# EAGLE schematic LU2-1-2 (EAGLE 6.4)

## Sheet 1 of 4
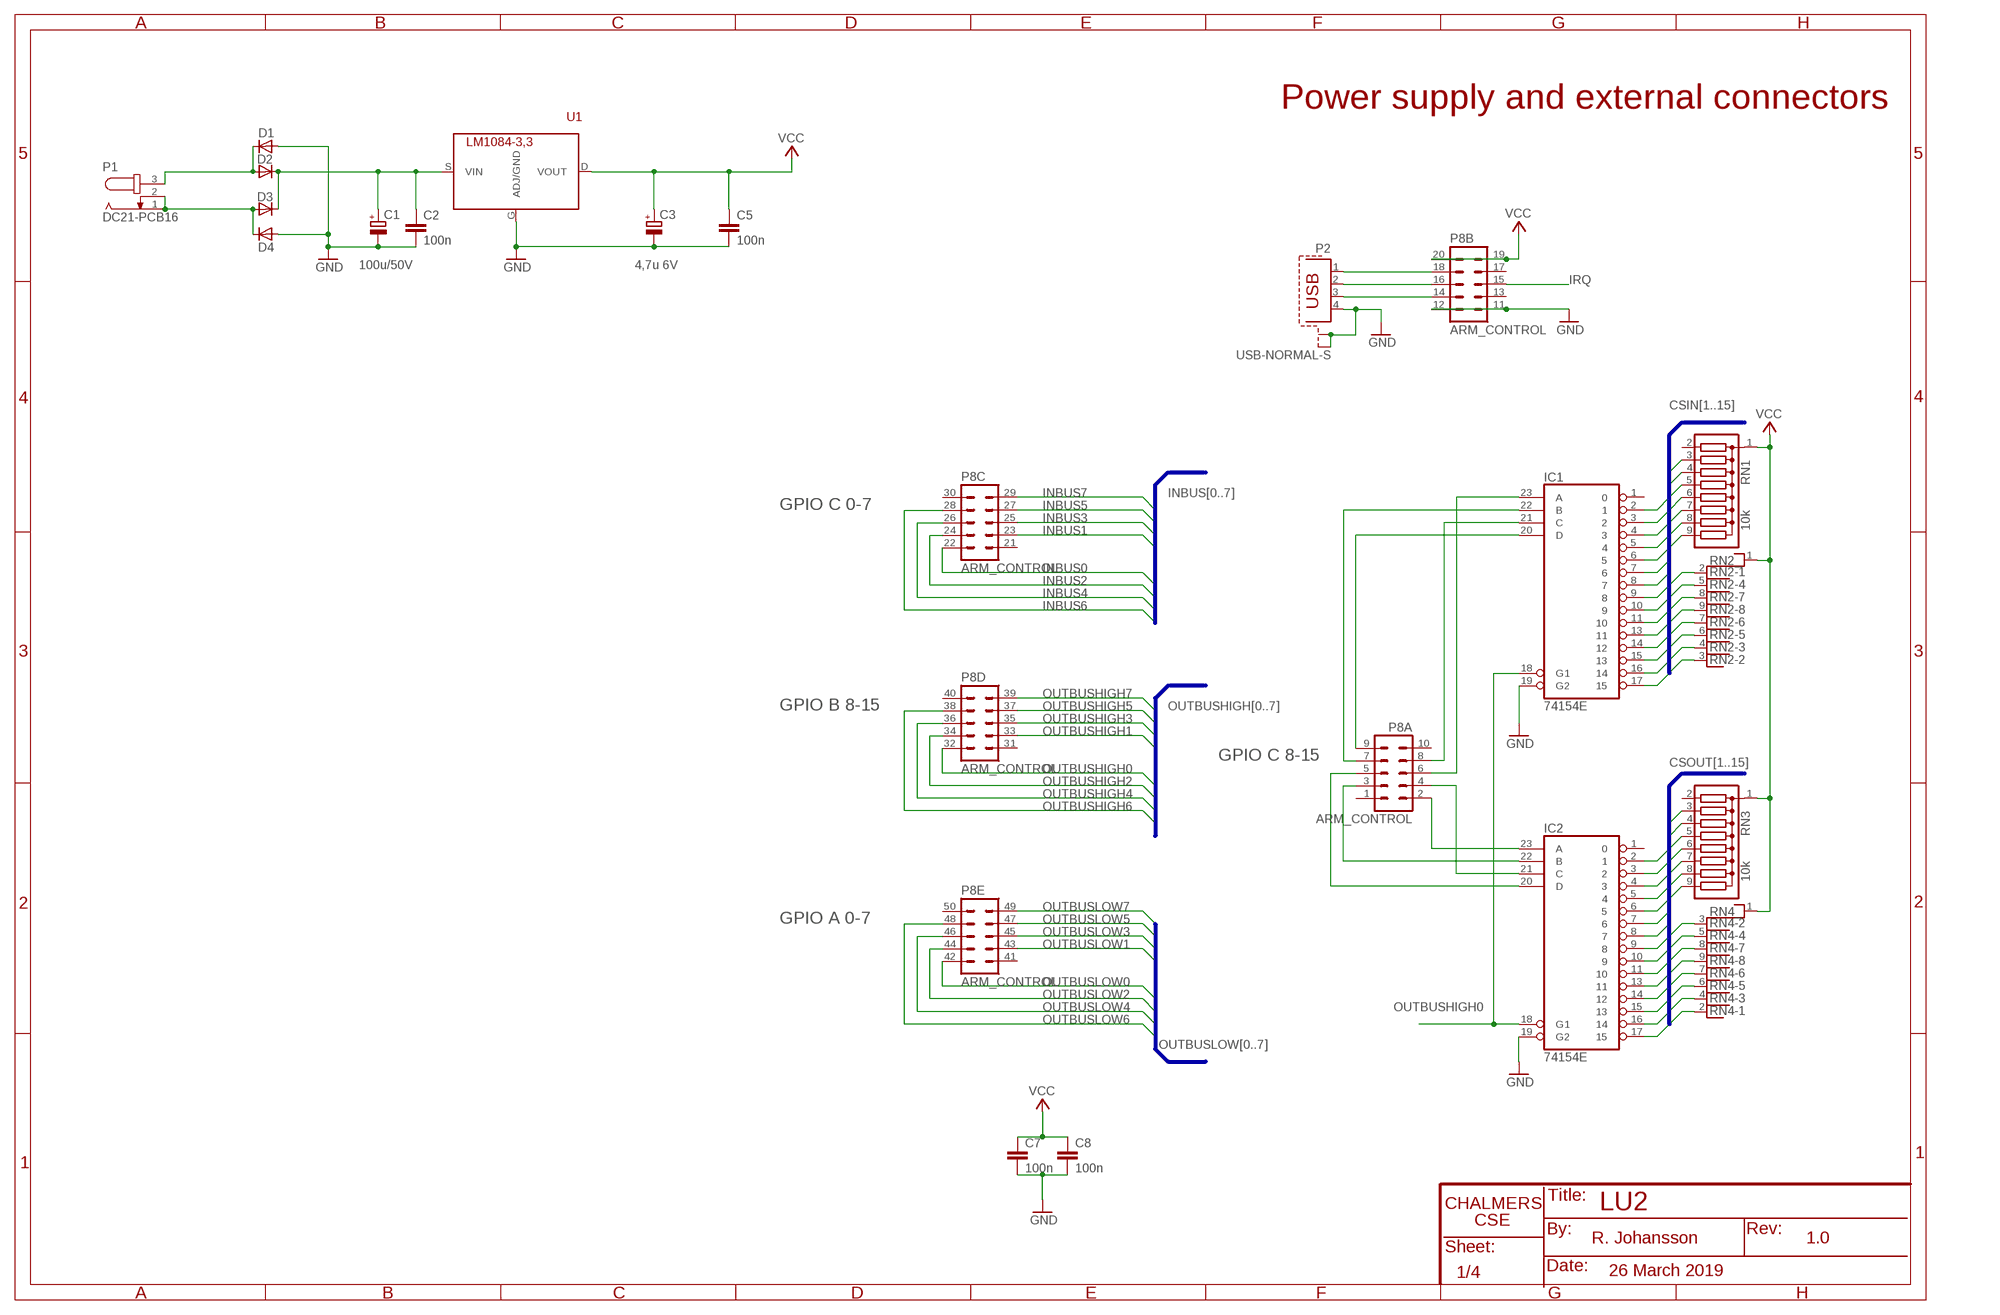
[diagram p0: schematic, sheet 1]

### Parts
C1  100u/50V  CPOL-EUE5-8.5  [E5-8,5]
C2  100n  C-EU050-024X044  [C050-024X044]
C3  4,7u 6V  CPOL-EUE5-5  [E5-5]
C5  100n  C-EU050-024X044  [C050-024X044]
C7  100n  C313  [C313]
C8  100n  C313  [C313]
D1  1N4004  [DO41-10]
D2  1N4004  [DO41-10]
D3  1N4004  [DO41-10]
D4  1N4004  [DO41-10]
IC1  74154E  [DIL24-3]
IC2  74154E  [DIL24-3]
P1  DC21-PCB16  [DC21CLIFF]
P2  USB-NORMAL-S  [1729-S]
P8  ARM_CONTROL  [ARM_CTRL]
RN1  10k  SIL9  [SIL9R]
RN2  RNX8  [RN-9]
RN3  10k  SIL9  [SIL9R]
RN4  RNX8  [RN-9]
U1  LM1084-3,3  LM1117T  [TO220AH]

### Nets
CSIN1: IC1.2 RN1.3 ; also sheet 4
CSIN2: IC1.3 RN1.4 ; also sheet 4
CSIN3: IC1.4 RN1.5 ; also sheet 4
CSIN4: IC1.5 RN1.6 ; also sheet 4
CSIN5: IC1.6 RN1.7 ; also sheet 3
CSIN6: IC1.7 RN1.8 ; also sheet 3
CSIN7: IC1.8 RN1.9 ; also sheet 3
CSIN8: IC1.9 RN2.2 ; also sheet 3
CSIN9: IC1.10 RN2.5 ; also sheet 2
CSIN10: IC1.11 RN2.8 ; also sheet 2
CSIN11: IC1.13 RN2.9
CSIN12: IC1.14 RN2.7
CSIN13: IC1.15 RN2.6
CSIN14: IC1.16 RN2.4
CSIN15: IC1.17 RN2.3
CSOUT1: IC2.2 RN3.3
CSOUT2: IC2.3 RN3.4
CSOUT3: IC2.4 RN3.5
CSOUT4: IC2.5 RN3.6
CSOUT5: IC2.6 RN3.7
CSOUT6: IC2.7 RN3.8
CSOUT7: IC2.8 RN3.9 ; also sheet 2
CSOUT8: IC2.9 RN4.3 ; also sheet 2
CSOUT9: IC2.10 RN4.5 ; also sheet 2
CSOUT10: IC2.11 RN4.8 ; also sheet 2
CSOUT11: IC2.13 RN4.9 ; also sheet 2
CSOUT12: IC2.14 RN4.7 ; also sheet 2
CSOUT13: IC2.15 RN4.6 ; also sheet 2
CSOUT14: IC2.16 RN4.4 ; also sheet 3
CSOUT15: IC2.17 RN4.2 ; also sheet 3
GND: C1.- C2.2 C3.- C5.2 C7.2 C8.2 D1.A D4.A IC1.19(G2) IC2.19(G2) P2.4 P2.S1 P2.S2 P8.11 P8.12 U1.G(ADJ/GND) ; also sheet 2,3,4
INBUS0: P8.22 ; also sheet 2,3
INBUS1: P8.23 ; also sheet 2,3
INBUS2: P8.24 ; also sheet 2,3
INBUS3: P8.25 ; also sheet 2,3
INBUS4: P8.26 ; also sheet 2,3
INBUS5: P8.27 ; also sheet 2,3
INBUS6: P8.28 ; also sheet 2,3
INBUS7: P8.29 ; also sheet 2,3
IRQ: P8.15 ; also sheet 3
N$29: IC1.21(C) P8.8
N$31: IC1.22(B) P8.7
N$33: IC1.23(A) P8.6
N$35: IC2.23(A) P8.2
N$37: IC2.22(B) P8.3
N$46: IC2.21(C) P8.4
N$47: IC2.20(D) P8.5
N$48: P2.1 P8.18
N$49: P2.2 P8.16
N$52: D3.A D4.C P1.1 P1.2
N$55: P2.3 P8.14
N$306: D1.C D2.A P1.3
N$307: C1.+ C2.1 D2.C D3.C U1.S(VIN)
N$342: IC1.20(D) P8.9
OUTBUSHIGH0: IC1.18(G1) IC2.18(G1) P8.32
OUTBUSHIGH1: P8.33 ; also sheet 2
OUTBUSHIGH2: P8.34 ; also sheet 4
OUTBUSHIGH3: P8.35 ; also sheet 4
OUTBUSHIGH4: P8.36 ; also sheet 4
OUTBUSHIGH5: P8.37 ; also sheet 4
OUTBUSHIGH6: P8.38
OUTBUSHIGH7: P8.39 ; also sheet 2
OUTBUSLOW0: P8.42 ; also sheet 2,3
OUTBUSLOW1: P8.43 ; also sheet 2,3
OUTBUSLOW2: P8.44 ; also sheet 2,3
OUTBUSLOW3: P8.45 ; also sheet 2,3
OUTBUSLOW4: P8.46 ; also sheet 2,3
OUTBUSLOW5: P8.47 ; also sheet 2,3
OUTBUSLOW6: P8.48 ; also sheet 2,3
OUTBUSLOW7: P8.49 ; also sheet 2,3
VCC: C3.+ C5.1 C7.1 C8.1 P8.19 P8.20 RN1.1 RN2.1 RN3.1 RN4.1 U1.D(VOUT) ; also sheet 2,3,4
Unconnected: IC1.1 IC2.1 P8.1 P8.10 P8.13 P8.17 P8.21 P8.30 P8.31 P8.40 P8.41 P8.50 RN1.2 RN3.2

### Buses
INBUS[0..7]
OUTBUSLOW[0..7]
OUTBUSHIGH[0..7]
CSOUT[1..15]
CSIN[1..15]

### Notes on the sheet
- Power supply and external connectors
- GPIO C 0-7
- GPIO B 8-15
- GPIO C 8-15
- GPIO A 0-7
- LU2
- 1.0
- R. Johansson
- 26 March 2019

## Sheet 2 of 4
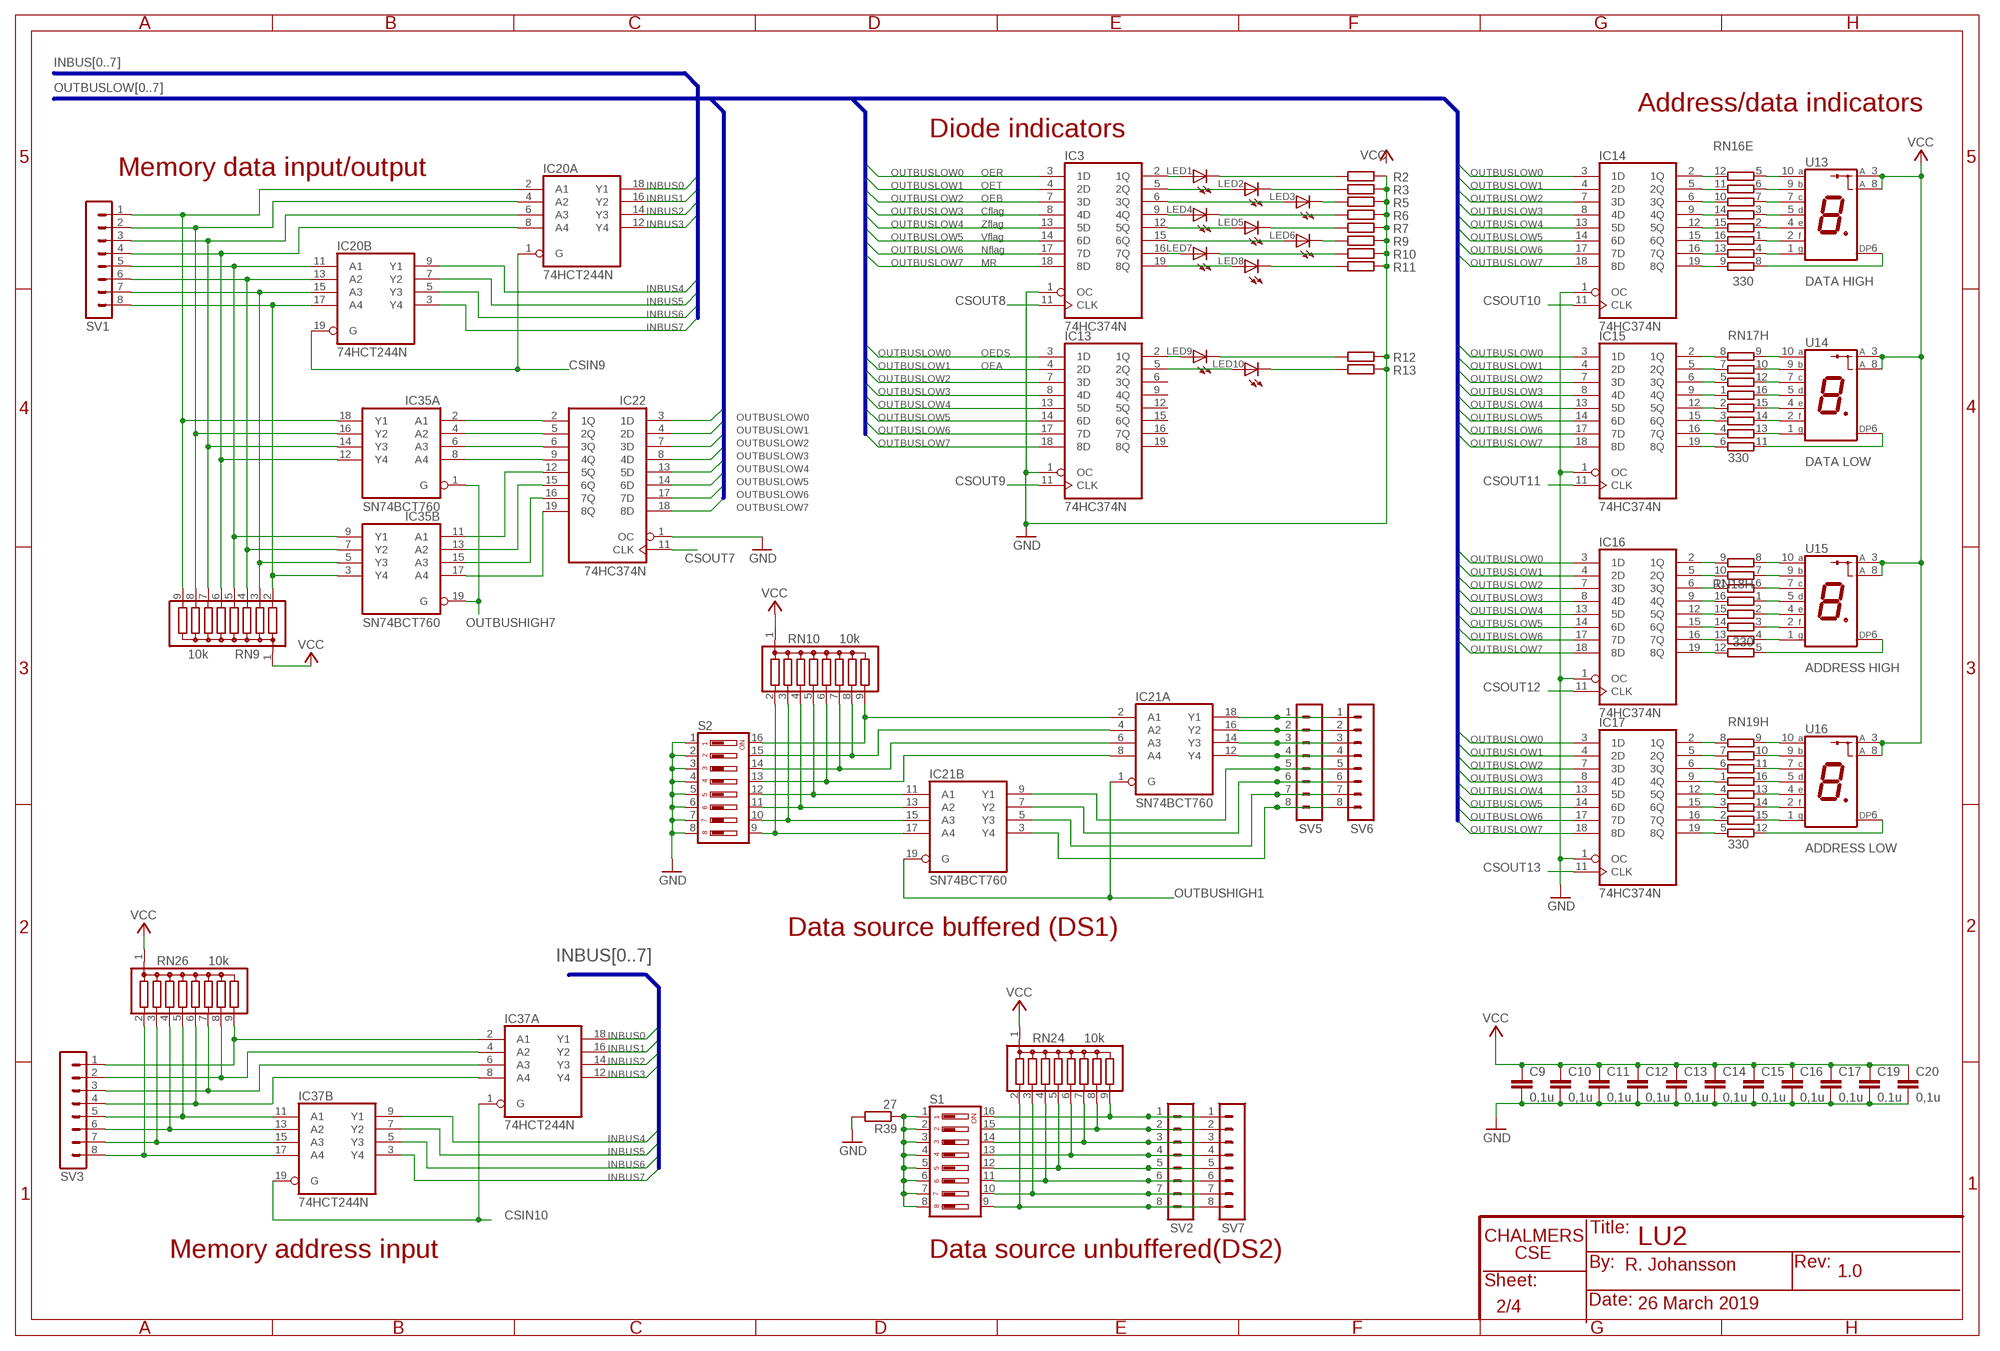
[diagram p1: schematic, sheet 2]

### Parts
C9  0,1u  C313  [C313]
C10  0,1u  C313  [C313]
C11  0,1u  C313  [C313]
C12  0,1u  C313  [C313]
C13  0,1u  C313  [C313]
C14  0,1u  C313  [C313]
C15  0,1u  C313  [C313]
C16  0,1u  C313  [C313]
C17  0,1u  C313  [C313]
C19  0,1u  C313  [C313]
C20  0,1u  C313  [C313]
IC3  74HC374N  [DIL20]
IC13  74HC374N  [DIL20]
IC14  74HC374N  [DIL20]
IC15  74HC374N  [DIL20]
IC16  74HC374N  [DIL20]
IC17  74HC374N  [DIL20]
IC20  74HCT244N  [DIL20]
IC21  SN74BCT760  74HCT244N  [DIL20]
IC22  74HC374N  [DIL20]
IC35  SN74BCT760  74HC244N  [DIL20]
IC37  74HCT244N  [DIL20]
LED1  RED  LED3MM  [LED3MM]
LED2  RED  LED3MM  [LED3MM]
LED3  RED  LED3MM  [LED3MM]
LED4  RED  LED3MM  [LED3MM]
LED5  RED  LED3MM  [LED3MM]
LED6  RED  LED3MM  [LED3MM]
LED7  RED  LED3MM  [LED3MM]
LED8  RED  LED3MM  [LED3MM]
LED9  RED  LED3MM  [LED3MM]
LED10  RED  LED3MM  [LED3MM]
R2  R-EU_0204/7  [0204/7]
R3  R-EU_0204/7  [0204/7]
R5  R-EU_0204/7  [0204/7]
R6  R-EU_0204/7  [0204/7]
R7  R-EU_0204/7  [0204/7]
R9  R-EU_0204/7  [0204/7]
R10  R-EU_0204/7  [0204/7]
R11  R-EU_0204/7  [0204/7]
R12  R-EU_0204/7  [0204/7]
R13  R-EU_0204/7  [0204/7]
R39  27  R-EU_0204/7  [0204/7]
RN9  10k  SIL9  [SIL9R]
RN10  10k  SIL9  [SIL9R]
RN16  330  8R-N  [DIL16]
RN17  330  8R-N  [DIL16]
RN18  330  8R-N  [DIL16]
RN19  330  8R-N  [DIL16]
RN24  10k  SIL9  [SIL9R]
RN26  10k  SIL9  [SIL9R]
S1  DS08  [DS-08]
S2  DS08  [DS-08]
SV1  MA08R-1  [MA08R-1]
SV2  MA08R-1  [MA08R-1]
SV3  MA08R-1  [MA08R-1]
SV5  MA08R-1  [MA08R-1]
SV6  MA08R-1  [MA08R-1]
SV7  MA08R-1  [MA08R-1]
U13  DATA HIGH  LED7_CA  [LED7SEG]
U14  DATA LOW  LED7_CA  [LED7SEG]
U15  ADDRESS HIGH  LED7_CA  [LED7SEG]
U16  ADDRESS LOW  LED7_CA  [LED7SEG]

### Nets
CSIN9: IC20.1(A:G) IC20.19(B:G) ; also sheet 1
CSIN10: IC37.1(A:G) IC37.19(B:G) ; also sheet 1
CSOUT7: IC22.11(CLK) ; also sheet 1
CSOUT8: IC3.11(CLK) ; also sheet 1
CSOUT9: IC13.11(CLK) ; also sheet 1
CSOUT10: IC14.11(CLK) ; also sheet 1
CSOUT11: IC15.11(CLK) ; also sheet 1
CSOUT12: IC16.11(CLK) ; also sheet 1
CSOUT13: IC17.11(CLK) ; also sheet 1
GND: C9.2 C10.2 C11.2 C12.2 C13.2 C14.2 C15.2 C16.2 C17.2 C19.2 C20.2 IC3.1(OC) IC13.1(OC) IC14.1(OC) IC15.1(OC) IC16.1(OC) IC17.1(OC) IC22.1(OC) R2.2 R3.2 R5.2 R6.2 R7.2 R9.2 R10.2 R11.2 R12.2 R13.2 R39.2 S2.1 S2.2 S2.3 S2.4 S2.5 S2.6 S2.7 S2.8 ; also sheet 1,3,4
INBUS0: IC20.18(A:Y1) IC37.18(A:Y1) ; also sheet 1,3
INBUS1: IC20.16(A:Y2) IC37.16(A:Y2) ; also sheet 1,3
INBUS2: IC20.14(A:Y3) IC37.14(A:Y3) ; also sheet 1,3
INBUS3: IC20.12(A:Y4) IC37.12(A:Y4) ; also sheet 1,3
INBUS4: IC20.9(B:Y1) IC37.9(B:Y1) ; also sheet 1,3
INBUS5: IC20.7(B:Y2) IC37.7(B:Y2) ; also sheet 1,3
INBUS6: IC20.5(B:Y3) IC37.5(B:Y3) ; also sheet 1,3
INBUS7: IC20.3(B:Y4) IC37.3(B:Y4) ; also sheet 1,3
N$1: IC13.2(1Q) LED9.A
N$3: IC13.5(2Q) LED10.A
N$4: IC3.19(8Q) LED8.A
N$5: IC3.16(7Q) LED7.A
N$7: IC22.19(8Q) IC35.17(B:A4)
N$8: LED1.K(C) R2.1
N$9: LED2.K(C) R3.1
N$10: LED3.K(C) R5.1
N$11: LED4.K(C) R6.1
N$12: LED5.K(C) R7.1
N$13: LED6.K(C) R9.1
N$14: LED7.K(C) R10.1
N$15: LED8.K(C) R11.1
N$16: IC3.15(6Q) LED6.A
N$17: IC3.12(5Q) LED5.A
N$18: IC20.17(B:A4) IC35.3(B:Y4) RN9.2 SV1.8
N$19: IC3.9(4Q) LED4.A
N$20: IC3.6(3Q) LED3.A
N$21: IC3.5(2Q) LED2.A
N$22: IC3.2(1Q) LED1.A
N$23: LED9.K(C) R12.1
N$24: LED10.K(C) R13.1
N$39: IC20.15(B:A3) IC35.5(B:Y3) RN9.3 SV1.7
N$78: IC20.13(B:A2) IC35.7(B:Y2) RN9.4 SV1.6
N$145: RN19.12 U16.6(DP)
N$146: RN19.15 U16.1(G)
N$147: RN19.14 U16.2(F)
N$148: RN19.13 U16.4(E)
N$149: RN19.16 U16.5(D)
N$150: RN19.11 U16.7(C)
N$151: RN19.10 U16.9(B)
N$152: RN19.9 U16.10(A)
N$153: IC17.19(8Q) RN19.5
N$154: IC17.16(7Q) RN19.2
N$155: IC17.15(6Q) RN19.3
N$156: IC17.12(5Q) RN19.4
N$157: IC17.9(4Q) RN19.1
N$158: IC17.6(3Q) RN19.6
N$159: IC17.5(2Q) RN19.7
N$160: IC17.2(1Q) RN19.8
N$161: RN18.5 U15.6(DP)
N$162: RN18.4 U15.1(G)
N$163: RN18.3 U15.2(F)
N$164: RN18.2 U15.4(E)
N$165: RN18.1 U15.5(D)
N$166: RN18.6 U15.7(C)
N$167: RN18.7 U15.9(B)
N$168: RN18.8 U15.10(A)
N$169: IC16.2(1Q) RN18.9
N$170: IC16.5(2Q) RN18.10
N$171: IC16.6(3Q) RN18.11
N$172: IC16.9(4Q) RN18.16
N$173: IC16.12(5Q) RN18.15
N$174: IC16.15(6Q) RN18.14
N$175: IC16.16(7Q) RN18.13
N$176: IC16.19(8Q) RN18.12
N$177: RN17.11 U14.6(DP)
N$178: RN17.13 U14.1(G)
N$179: RN17.14 U14.2(F)
N$180: RN17.15 U14.4(E)
N$181: RN17.16 U14.5(D)
N$182: RN17.12 U14.7(C)
N$183: RN17.10 U14.9(B)
N$184: RN17.9 U14.10(A)
N$185: IC15.19(8Q) RN17.6
N$186: IC15.16(7Q) RN17.4
N$187: IC15.15(6Q) RN17.3
N$188: IC15.12(5Q) RN17.2
N$189: IC15.9(4Q) RN17.1
N$190: IC15.6(3Q) RN17.5
N$191: IC15.5(2Q) RN17.7
N$192: IC15.2(1Q) RN17.8
N$197: IC14.2(1Q) RN16.12
N$198: IC14.5(2Q) RN16.11
N$199: IC14.6(3Q) RN16.10
N$200: IC14.9(4Q) RN16.14
N$201: IC14.12(5Q) RN16.15
N$202: IC14.15(6Q) RN16.16
N$203: IC14.16(7Q) RN16.13
N$204: IC14.19(8Q) RN16.9
N$213: RN16.5 U13.10(A)
N$214: RN16.6 U13.9(B)
N$215: RN16.7 U13.7(C)
N$216: RN16.3 U13.5(D)
N$217: RN16.2 U13.4(E)
N$218: RN16.1 U13.2(F)
N$219: RN16.4 U13.1(G)
N$220: RN16.8 U13.6(DP)
N$230: IC20.11(B:A1) IC35.9(B:Y1) RN9.5 SV1.5
N$248: IC20.8(A:A4) IC35.12(A:Y4) RN9.6 SV1.4
N$283: IC20.6(A:A3) IC35.14(A:Y3) RN9.7 SV1.3
N$284: IC20.4(A:A2) IC35.16(A:Y2) RN9.8 SV1.2
N$285: IC20.2(A:A1) IC35.18(A:Y1) RN9.9 SV1.1
N$287: IC21.17(B:A4) RN10.2 S2.9
N$288: IC21.15(B:A3) RN10.3 S2.10
N$289: IC21.13(B:A2) RN10.4 S2.11
N$290: IC21.11(B:A1) RN10.5 S2.12
N$291: IC21.8(A:A4) RN10.6 S2.13
N$292: IC21.6(A:A3) RN10.7 S2.14
N$293: IC21.4(A:A2) RN10.8 S2.15
N$294: IC21.2(A:A1) RN10.9 S2.16
N$358: IC22.16(7Q) IC35.15(B:A3)
N$359: IC22.15(6Q) IC35.13(B:A2)
N$360: IC22.12(5Q) IC35.11(B:A1)
N$361: IC22.9(4Q) IC35.8(A:A4)
N$362: IC22.6(3Q) IC35.6(A:A3)
N$363: IC22.5(2Q) IC35.4(A:A2)
N$364: IC22.2(1Q) IC35.2(A:A1)
N$381: R39.1 S1.1 S1.2 S1.3 S1.4 S1.5 S1.6 S1.7 S1.8
N$382: RN24.2 S1.9 SV2.8 SV7.8
N$383: RN24.3 S1.10 SV2.7 SV7.7
N$384: RN24.4 S1.11 SV2.6 SV7.6
N$385: RN24.5 S1.12 SV2.5 SV7.5
N$387: RN24.7 S1.14 SV2.3 SV7.3
N$388: RN24.8 S1.15 SV2.2 SV7.2
N$397: IC37.17(B:A4) RN26.2 SV3.8
N$406: IC37.15(B:A3) RN26.3 SV3.7
N$407: IC37.13(B:A2) RN26.4 SV3.6
N$408: IC37.11(B:A1) RN26.5 SV3.5
N$409: IC37.8(A:A4) RN26.6 SV3.4
N$412: IC37.6(A:A3) RN26.7 SV3.3
N$413: IC37.4(A:A2) RN26.8 SV3.2
N$419: RN24.9 S1.16 SV2.1 SV7.1
N$420: RN24.6 S1.13 SV2.4 SV7.4
N$436: IC37.2(A:A1) RN26.9 SV3.1
OUTBUSHIGH1: IC21.1(A:G) IC21.19(B:G) ; also sheet 1
OUTBUSHIGH7: IC35.1(A:G) IC35.19(B:G) ; also sheet 1
OUTBUSLOW0: IC3.3(1D) IC13.3(1D) IC14.3(1D) IC15.3(1D) IC16.3(1D) IC17.3(1D) IC22.3(1D) ; also sheet 1,3
OUTBUSLOW1: IC3.4(2D) IC13.4(2D) IC14.4(2D) IC15.4(2D) IC16.4(2D) IC17.4(2D) IC22.4(2D) ; also sheet 1,3
OUTBUSLOW2: IC3.7(3D) IC13.7(3D) IC14.7(3D) IC15.7(3D) IC16.7(3D) IC17.7(3D) IC22.7(3D) ; also sheet 1,3
OUTBUSLOW3: IC3.8(4D) IC13.8(4D) IC14.8(4D) IC15.8(4D) IC16.8(4D) IC17.8(4D) IC22.8(4D) ; also sheet 1,3
OUTBUSLOW4: IC3.13(5D) IC13.13(5D) IC14.13(5D) IC15.13(5D) IC16.13(5D) IC17.13(5D) IC22.13(5D) ; also sheet 1,3
OUTBUSLOW5: IC3.14(6D) IC13.14(6D) IC14.14(6D) IC15.14(6D) IC16.14(6D) IC17.14(6D) IC22.14(6D) ; also sheet 1,3
OUTBUSLOW6: IC3.17(7D) IC13.17(7D) IC14.17(7D) IC15.17(7D) IC16.17(7D) IC17.17(7D) IC22.17(7D) ; also sheet 1,3
OUTBUSLOW7: IC3.18(8D) IC13.18(8D) IC14.18(8D) IC15.18(8D) IC16.18(8D) IC17.18(8D) IC22.18(8D) ; also sheet 1,3
OUTBUSLOW8: IC21.18(A:Y1) SV5.1 SV6.1
OUTBUSLOW9: IC21.16(A:Y2) SV5.2 SV6.2
OUTBUSLOW10: IC21.14(A:Y3) SV5.3 SV6.3
OUTBUSLOW11: IC21.12(A:Y4) SV5.4 SV6.4
OUTBUSLOW12: IC21.9(B:Y1) SV5.5 SV6.5
OUTBUSLOW13: IC21.7(B:Y2) SV5.6 SV6.6
OUTBUSLOW14: IC21.5(B:Y3) SV5.7 SV6.7
OUTBUSLOW15: IC21.3(B:Y4) SV5.8 SV6.8
VCC: C9.1 C10.1 C11.1 C12.1 C13.1 C14.1 C15.1 C16.1 C17.1 C19.1 C20.1 RN9.1 RN10.1 RN24.1 RN26.1 U13.3(A) U13.8(A) U14.3(A) U14.8(A) U15.3(A) U15.8(A) U16.3(A) U16.8(A) ; also sheet 1,3,4
Unconnected: IC13.6(3Q) IC13.9(4Q) IC13.12(5Q) IC13.15(6Q) IC13.16(7Q) IC13.19(8Q)

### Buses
OUTBUSLOW[0..7]
INBUS[0..7]

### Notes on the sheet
- Address/data indicators
- Diode indicators
- Memory data input/output | OER
- OET
- OEB
- Cflag
- Zflag
- Vflag
- Nflag
- MR
- OEDS
- OEA
- Data source buffered (DS1)
- LU2
- Memory address input | Data source unbuffered(DS2)
- R. Johansson
- 1.0
- 26 March 2019

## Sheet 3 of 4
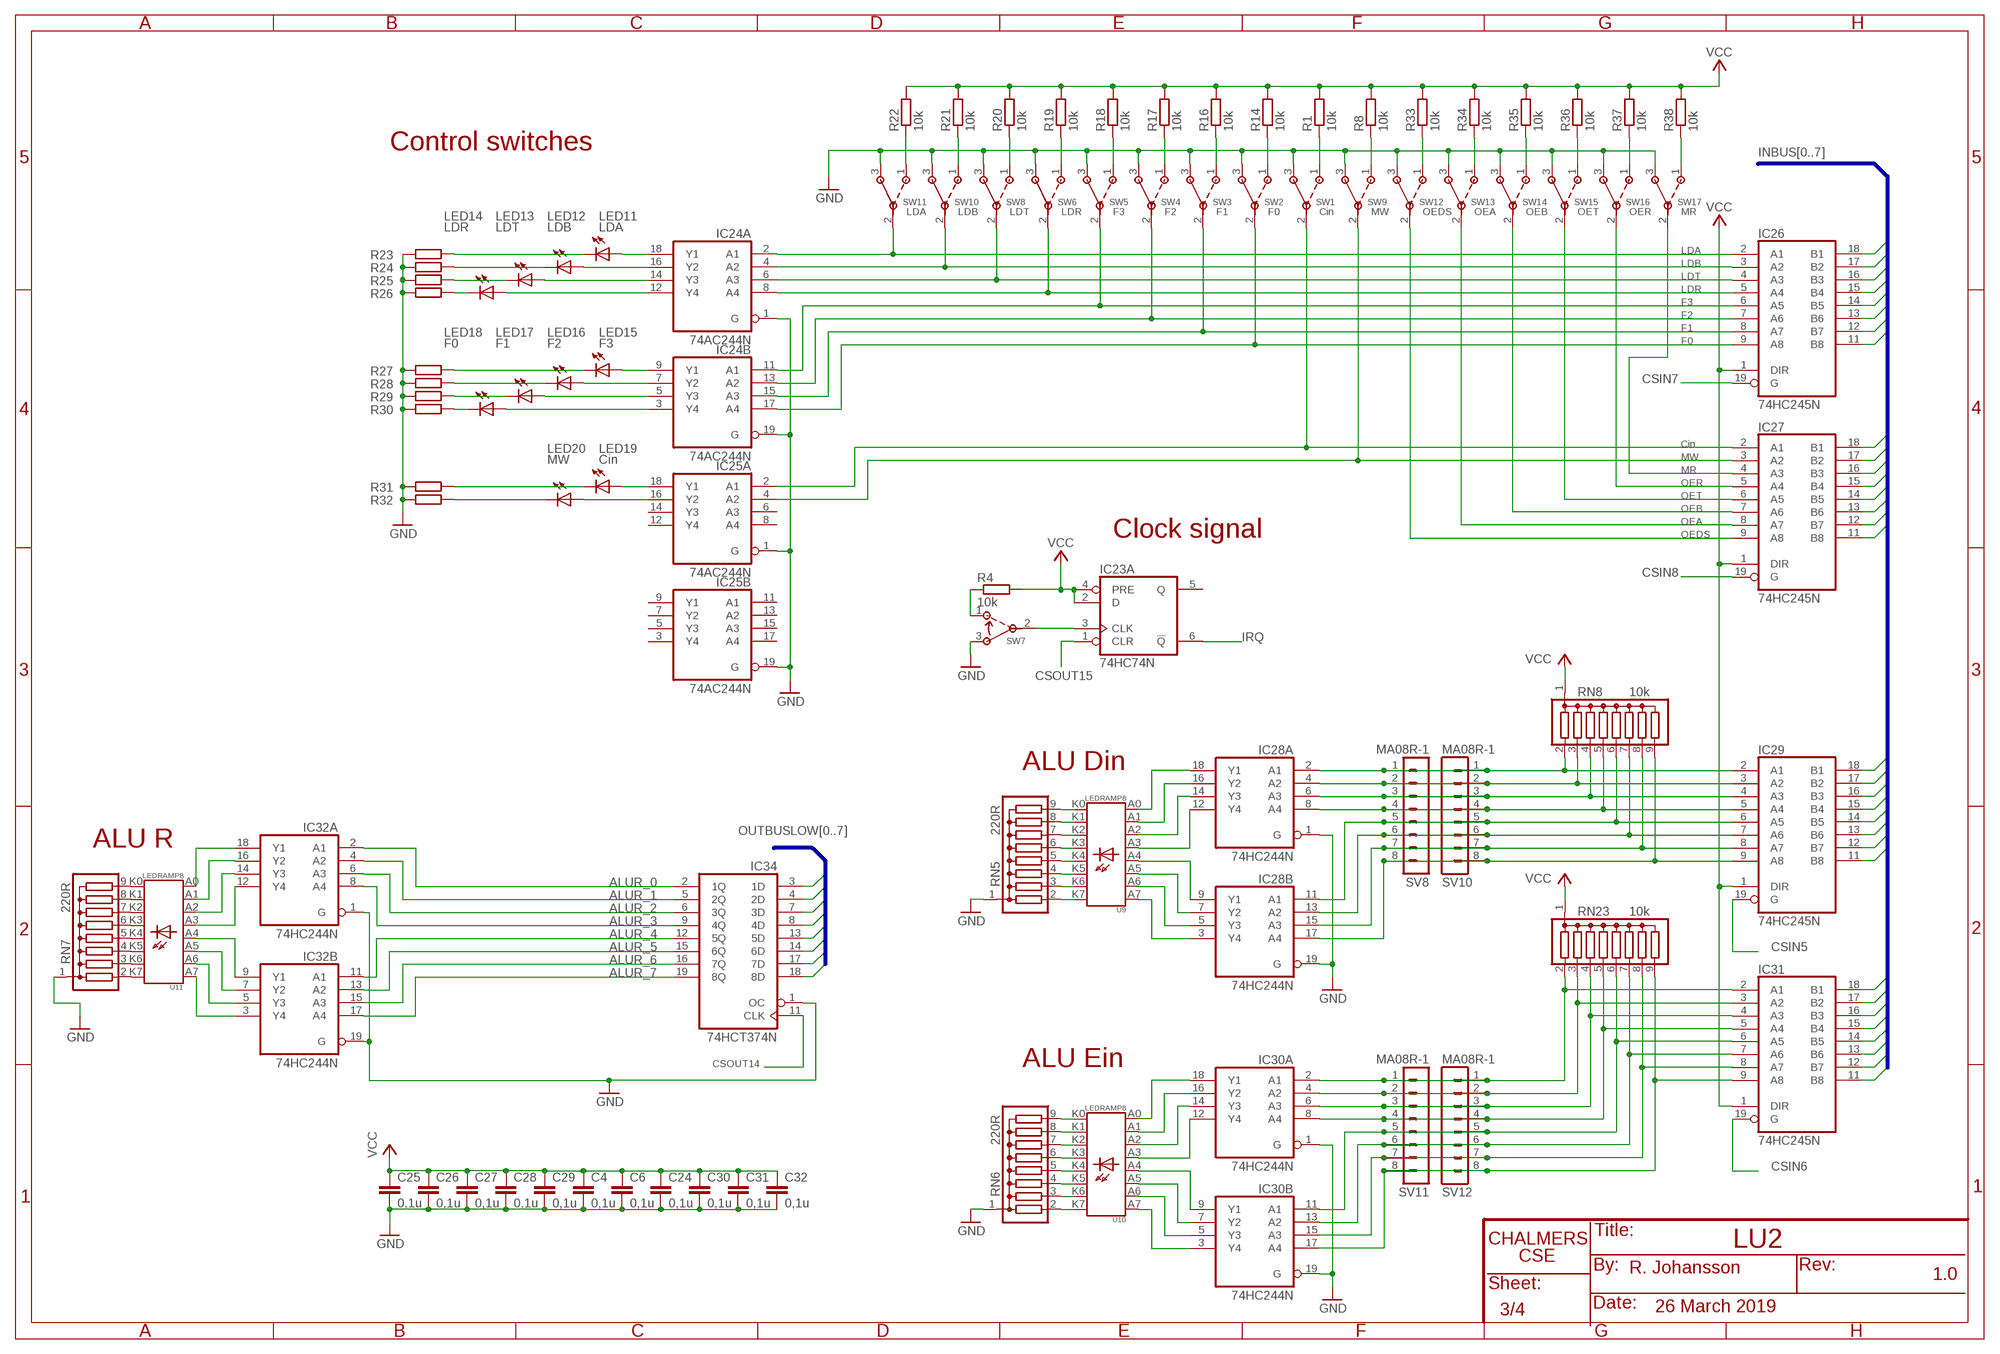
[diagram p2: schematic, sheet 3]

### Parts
C4  0,1u  C313  [C313]
C6  0,1u  C313  [C313]
C24  0,1u  C313  [C313]
C25  0,1u  C313  [C313]
C26  0,1u  C313  [C313]
C27  0,1u  C313  [C313]
C28  0,1u  C313  [C313]
C29  0,1u  C313  [C313]
C30  0,1u  C313  [C313]
C31  0,1u  C313  [C313]
C32  0,1u  C313  [C313]
IC23  74HC74N  [DIL14]
IC24  74AC244N  [DIL20]
IC25  74AC244N  [DIL20]
IC26  74HC245N  [DIL20]
IC27  74HC245N  [DIL20]
IC28  74HC244N  [DIL20]
IC29  74HC245N  [DIL20]
IC30  74HC244N  [DIL20]
IC31  74HC245N  [DIL20]
IC32  74HC244N  [DIL20]
IC34  74HCT374N  [DIL20]
LED11  LDA  LED3MM  [LED3MM]
LED12  LDB  LED3MM  [LED3MM]
LED13  LDT  LED3MM  [LED3MM]
LED14  LDR  LED3MM  [LED3MM]
LED15  F3  LED3MM  [LED3MM]
LED16  F2  LED3MM  [LED3MM]
LED17  F1  LED3MM  [LED3MM]
LED18  F0  LED3MM  [LED3MM]
LED19  Cin  LED3MM  [LED3MM]
LED20  MW  LED3MM  [LED3MM]
R1  10k  R-EU_0204/7  [0204/7]
R4  10k  R-EU_0207/7  [0207/7]
R8  10k  R-EU_0204/7  [0204/7]
R14  10k  R-EU_0204/7  [0204/7]
R16  10k  R-EU_0204/7  [0204/7]
R17  10k  R-EU_0204/7  [0204/7]
R18  10k  R-EU_0204/7  [0204/7]
R19  10k  R-EU_0204/7  [0204/7]
R20  10k  R-EU_0204/7  [0204/7]
R21  10k  R-EU_0204/7  [0204/7]
R22  10k  R-EU_0204/7  [0204/7]
R23  R-EU_0204/7  [0204/7]
R24  R-EU_0204/7  [0204/7]
R25  R-EU_0204/7  [0204/7]
R26  R-EU_0204/7  [0204/7]
R27  R-EU_0204/7  [0204/7]
R28  R-EU_0204/7  [0204/7]
R29  R-EU_0204/7  [0204/7]
R30  R-EU_0204/7  [0204/7]
R31  R-EU_0204/7  [0204/7]
R32  R-EU_0204/7  [0204/7]
R33  10k  R-EU_0204/7  [0204/7]
R34  10k  R-EU_0204/7  [0204/7]
R35  10k  R-EU_0204/7  [0204/7]
R36  10k  R-EU_0204/7  [0204/7]
R37  10k  R-EU_0204/7  [0204/7]
R38  10k  R-EU_0204/7  [0204/7]
RN5  220R  SIL9  [SIL9R]
RN6  220R  SIL9  [SIL9R]
RN7  220R  SIL9  [SIL9R]
RN8  10k  SIL9  [SIL9R]
RN23  10k  SIL9  [SIL9R]
SV8  MA08R-1  [MA08R-1]
SV10  MA08R-1  [MA08R-1]
SV11  MA08R-1  [MA08R-1]
SV12  MA08R-1  [MA08R-1]
SW1  ELEDIS_TOGGLE_MINIATURESMALL  [SWITCH_DV]
SW2  ELEDIS_TOGGLE_MINIATURESMALL  [SWITCH_DV]
SW3  ELEDIS_TOGGLE_MINIATURESMALL  [SWITCH_DV]
SW4  ELEDIS_TOGGLE_MINIATURESMALL  [SWITCH_DV]
SW5  ELEDIS_TOGGLE_MINIATURESMALL  [SWITCH_DV]
SW6  ELEDIS_TOGGLE_MINIATURESMALL  [SWITCH_DV]
SW7  ELEDIS_TOGGLE_MINIATURE_MOMSMALL  [SWITCH_DV]
SW8  ELEDIS_TOGGLE_MINIATURESMALL  [SWITCH_DV]
SW9  ELEDIS_TOGGLE_MINIATURESMALL  [SWITCH_DV]
SW10  ELEDIS_TOGGLE_MINIATURESMALL  [SWITCH_DV]
SW11  ELEDIS_TOGGLE_MINIATURESMALL  [SWITCH_DV]
SW12  ELEDIS_TOGGLE_MINIATURESMALL  [SWITCH_DV]
SW13  ELEDIS_TOGGLE_MINIATURESMALL  [SWITCH_DV]
SW14  ELEDIS_TOGGLE_MINIATURESMALL  [SWITCH_DV]
SW15  ELEDIS_TOGGLE_MINIATURESMALL  [SWITCH_DV]
SW16  ELEDIS_TOGGLE_MINIATURESMALL  [SWITCH_DV]
SW17  ELEDIS_TOGGLE_MINIATURESMALL  [SWITCH_DV]
U9  LEDRAMP8  [LEDRAMP8]
U10  LEDRAMP8  [LEDRAMP8]
U11  LEDRAMP8  [LEDRAMP8]

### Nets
ALUR_0: IC32.2(A:A1) IC34.2(1Q) ; also sheet 4
ALUR_1: IC32.4(A:A2) IC34.5(2Q) ; also sheet 4
ALUR_2: IC32.6(A:A3) IC34.6(3Q) ; also sheet 4
ALUR_3: IC32.8(A:A4) IC34.9(4Q) ; also sheet 4
ALUR_4: IC32.11(B:A1) IC34.12(5Q) ; also sheet 4
ALUR_5: IC32.13(B:A2) IC34.15(6Q) ; also sheet 4
ALUR_6: IC32.15(B:A3) IC34.16(7Q) ; also sheet 4
ALUR_7: IC32.17(B:A4) IC34.19(8Q) ; also sheet 4
CSIN5: IC29.19(G) ; also sheet 1
CSIN6: IC31.19(G) ; also sheet 1
CSIN7: IC26.19(G) ; also sheet 1
CSIN8: IC27.19(G) ; also sheet 1
CSOUT14: IC34.11(CLK) ; also sheet 1
CSOUT15: IC23.1(A:CLR) ; also sheet 1
GND: C4.2 C6.2 C24.2 C25.2 C26.2 C27.2 C28.2 C29.2 C30.2 C31.2 C32.2 IC24.1(A:G) IC24.19(B:G) IC25.1(A:G) IC25.19(B:G) IC28.1(A:G) IC28.19(B:G) IC30.1(A:G) IC30.19(B:G) IC32.1(A:G) IC32.19(B:G) IC34.1(OC) R23.1 R24.1 R25.1 R26.1 R27.1 R28.1 R29.1 R30.1 R31.1 R32.1 RN5.1 RN6.1 RN7.1 SW1.3 SW2.3 SW3.3 SW4.3 SW5.3 SW6.3 SW7.3 SW8.3 SW9.3 SW10.3 SW11.3 SW12.3 SW13.3 SW14.3 SW15.3 SW16.3 SW17.3 ; also sheet 1,2,4
INBUS0: IC26.18(B1) IC27.18(B1) IC29.18(B1) IC31.18(B1) ; also sheet 1,2
INBUS1: IC26.17(B2) IC27.17(B2) IC29.17(B2) IC31.17(B2) ; also sheet 1,2
INBUS2: IC26.16(B3) IC27.16(B3) IC29.16(B3) IC31.16(B3) ; also sheet 1,2
INBUS3: IC26.15(B4) IC27.15(B4) IC29.15(B4) IC31.15(B4) ; also sheet 1,2
INBUS4: IC26.14(B5) IC27.14(B5) IC29.14(B5) IC31.14(B5) ; also sheet 1,2
INBUS5: IC26.13(B6) IC27.13(B6) IC29.13(B6) IC31.13(B6) ; also sheet 1,2
INBUS6: IC26.12(B7) IC27.12(B7) IC29.12(B7) IC31.12(B7) ; also sheet 1,2
INBUS7: IC26.11(B8) IC27.11(B8) IC29.11(B8) IC31.11(B8) ; also sheet 1,2
IRQ: IC23.6(A:!Q) ; also sheet 1
N$2: IC27.9(A8) SW12.2
N$75: LED14.K(C) R26.2
N$90: RN5.9 U9.K0(C0)
N$91: RN5.8 U9.K1(C1)
N$101: RN5.7 U9.K2(C2)
N$102: IC24.2(A:A1) IC26.2(A1) SW11.2
N$103: LED13.K(C) R25.2
N$104: LED12.K(C) R24.2
N$117: LED11.K(C) R23.2
N$118: IC24.12(A:Y4) LED14.A
N$119: IC24.14(A:Y3) LED13.A
N$121: IC24.16(A:Y2) LED12.A
N$133: RN5.6 U9.K3(C3)
N$136: IC24.18(A:Y1) LED11.A
N$137: LED15.K(C) R27.2
N$138: LED16.K(C) R28.2
N$144: LED17.K(C) R29.2
N$238: LED18.K(C) R30.2
N$255: RN5.5 U9.K4(C4)
N$275: IC24.9(B:Y1) LED15.A
N$295: IC27.8(A7) SW13.2
N$296: IC24.7(B:Y2) LED16.A
N$297: IC27.7(A6) SW14.2
N$298: IC27.6(A5) SW15.2
N$299: IC24.5(B:Y3) LED17.A
N$300: R22.1 SW11.1
N$301: R21.1 SW10.1
N$302: R20.1 SW8.1
N$303: R19.1 SW6.1
N$304: R18.1 SW5.1
N$305: R17.1 SW4.1
N$308: IC24.3(B:Y4) LED18.A
N$309: RN5.4 U9.K5(C5)
N$310: R16.1 SW3.1
N$311: R14.1 SW2.1
N$312: R1.1 SW1.1
N$313: R8.1 SW9.1
N$314: LED19.K(C) R31.2
N$315: IC25.18(A:Y1) LED19.A
N$316: LED20.K(C) R32.2
N$317: IC25.16(A:Y2) LED20.A
N$318: IC24.4(A:A2) IC26.3(A2) SW10.2
N$319: RN5.3 U9.K6(C6)
N$320: IC24.6(A:A3) IC26.4(A3) SW8.2
N$321: IC24.8(A:A4) IC26.5(A4) SW6.2
N$322: RN5.2 U9.K7(C7)
N$323: IC28.12(A:Y4) U9.A3
N$324: IC28.14(A:Y3) U9.A2
N$325: IC28.16(A:Y2) U9.A1
N$326: IC24.11(B:A1) IC26.6(A5) SW5.2
N$327: IC24.13(B:A2) IC26.7(A6) SW4.2
N$328: IC24.15(B:A3) IC26.8(A7) SW3.2
N$329: IC24.17(B:A4) IC26.9(A8) SW2.2
N$330: IC25.2(A:A1) IC27.2(A1) SW1.2
N$331: IC25.4(A:A2) IC27.3(A2) SW9.2
N$332: IC27.5(A4) SW16.2
N$333: IC27.4(A3) SW17.2
N$334: IC28.18(A:Y1) U9.A0
N$335: IC28.9(B:Y1) U9.A4
N$336: IC28.7(B:Y2) U9.A5
N$337: IC28.5(B:Y3) U9.A6
N$338: IC28.3(B:Y4) U9.A7
N$339: R4.1 SW7.1
N$343: IC30.4(A:A2) IC31.3(A2) RN23.3 SV11.2 SV12.2
N$344: IC30.6(A:A3) IC31.4(A3) RN23.4 SV11.3 SV12.3
N$345: IC30.8(A:A4) IC31.5(A4) RN23.5 SV11.4 SV12.4
N$346: IC30.11(B:A1) IC31.6(A5) RN23.6 SV11.5 SV12.5
N$347: IC30.13(B:A2) IC31.7(A6) RN23.7 SV11.6 SV12.6
N$348: IC30.15(B:A3) IC31.8(A7) RN23.8 SV11.7 SV12.7
N$350: IC23.3(A:CLK) SW7.2
N$356: IC30.17(B:A4) IC31.9(A8) RN23.9 SV11.8 SV12.8
N$357: IC30.2(A:A1) IC31.2(A1) RN23.2 SV11.1 SV12.1
N$365: RN6.9 U10.K0(C0)
N$366: RN6.8 U10.K1(C1)
N$367: RN6.7 U10.K2(C2)
N$368: RN6.6 U10.K3(C3)
N$369: RN6.5 U10.K4(C4)
N$370: RN6.4 U10.K5(C5)
N$371: RN6.3 U10.K6(C6)
N$372: RN6.2 U10.K7(C7)
N$373: IC30.12(A:Y4) U10.A3
N$374: IC30.14(A:Y3) U10.A2
N$375: IC30.16(A:Y2) U10.A1
N$376: IC30.18(A:Y1) U10.A0
N$377: IC30.9(B:Y1) U10.A4
N$378: IC30.7(B:Y2) U10.A5
N$379: IC30.5(B:Y3) U10.A6
N$380: IC30.3(B:Y4) U10.A7
N$386: IC28.11(B:A1) IC29.6(A5) RN8.6 SV8.5 SV10.5
N$389: R38.1 SW17.1
N$398: RN7.9 U11.K0(C0)
N$399: RN7.8 U11.K1(C1)
N$400: RN7.7 U11.K2(C2)
N$401: RN7.6 U11.K3(C3)
N$402: RN7.5 U11.K4(C4)
N$403: RN7.4 U11.K5(C5)
N$404: RN7.3 U11.K6(C6)
N$405: RN7.2 U11.K7(C7)
N$414: R37.1 SW16.1
N$415: R36.1 SW15.1
N$416: R35.1 SW14.1
N$417: R34.1 SW13.1
N$418: R33.1 SW12.1
N$421: IC28.13(B:A2) IC29.7(A6) RN8.7 SV8.6 SV10.6
N$422: IC28.15(B:A3) IC29.8(A7) RN8.8 SV8.7 SV10.7
N$423: IC28.17(B:A4) IC29.9(A8) RN8.9 SV8.8 SV10.8
N$424: IC28.8(A:A4) IC29.5(A4) RN8.5 SV8.4 SV10.4
N$425: IC28.6(A:A3) IC29.4(A3) RN8.4 SV8.3 SV10.3
N$426: IC28.4(A:A2) IC29.3(A2) RN8.3 SV8.2 SV10.2
N$427: IC28.2(A:A1) IC29.2(A1) RN8.2 SV8.1 SV10.1
N$428: IC32.18(A:Y1) U11.A0
N$429: IC32.16(A:Y2) U11.A1
N$430: IC32.14(A:Y3) U11.A2
N$431: IC32.12(A:Y4) U11.A3
N$432: IC32.9(B:Y1) U11.A4
N$433: IC32.7(B:Y2) U11.A5
N$434: IC32.5(B:Y3) U11.A6
N$435: IC32.3(B:Y4) U11.A7
OUTBUSLOW0: IC34.3(1D) ; also sheet 1,2
OUTBUSLOW1: IC34.4(2D) ; also sheet 1,2
OUTBUSLOW2: IC34.7(3D) ; also sheet 1,2
OUTBUSLOW3: IC34.8(4D) ; also sheet 1,2
OUTBUSLOW4: IC34.13(5D) ; also sheet 1,2
OUTBUSLOW5: IC34.14(6D) ; also sheet 1,2
OUTBUSLOW6: IC34.17(7D) ; also sheet 1,2
OUTBUSLOW7: IC34.18(8D) ; also sheet 1,2
VCC: C4.1 C6.1 C24.1 C25.1 C26.1 C27.1 C28.1 C29.1 C30.1 C31.1 C32.1 IC23.2(A:D) IC23.4(A:PRE) IC26.1(DIR) IC27.1(DIR) IC29.1(DIR) IC31.1(DIR) R1.2 R4.2 R8.2 R14.2 R16.2 R17.2 R18.2 R19.2 R20.2 R21.2 R22.2 R33.2 R34.2 R35.2 R36.2 R37.2 R38.2 RN8.1 RN23.1 ; also sheet 1,2,4
Unconnected: IC23.5(A:Q) IC23.8(B:!Q) IC23.9(B:Q) IC23.10(B:PRE) IC23.11(B:CLK) IC23.12(B:D) IC23.13(B:CLR) IC25.3(B:Y4) IC25.5(B:Y3) IC25.6(A:A3) IC25.7(B:Y2) IC25.8(A:A4) IC25.9(B:Y1) IC25.11(B:A1) IC25.12(A:Y4) IC25.13(B:A2) IC25.14(A:Y3) IC25.15(B:A3) IC25.17(B:A4)

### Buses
INBUS[0..7]
OUTBUSLOW[0..7]

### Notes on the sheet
- Control switches
- LDA | LDB | LDT | LDR | F3 | F2 | F1 | F0 | Cin | MW | OEDS | OEA | OEB | OET | OER | MR
- LDA
- LDB
- LDT
- LDR
- F3
- F2
- F1
- F0
- Cin
- MW
- MR
- OER
- OET
- OEB
- OEA
- Clock signal | OEDS
- ALU Din
- ALU R
- ALU Ein
- LU2
- R. Johansson
- 1.0
- 26 March 2019

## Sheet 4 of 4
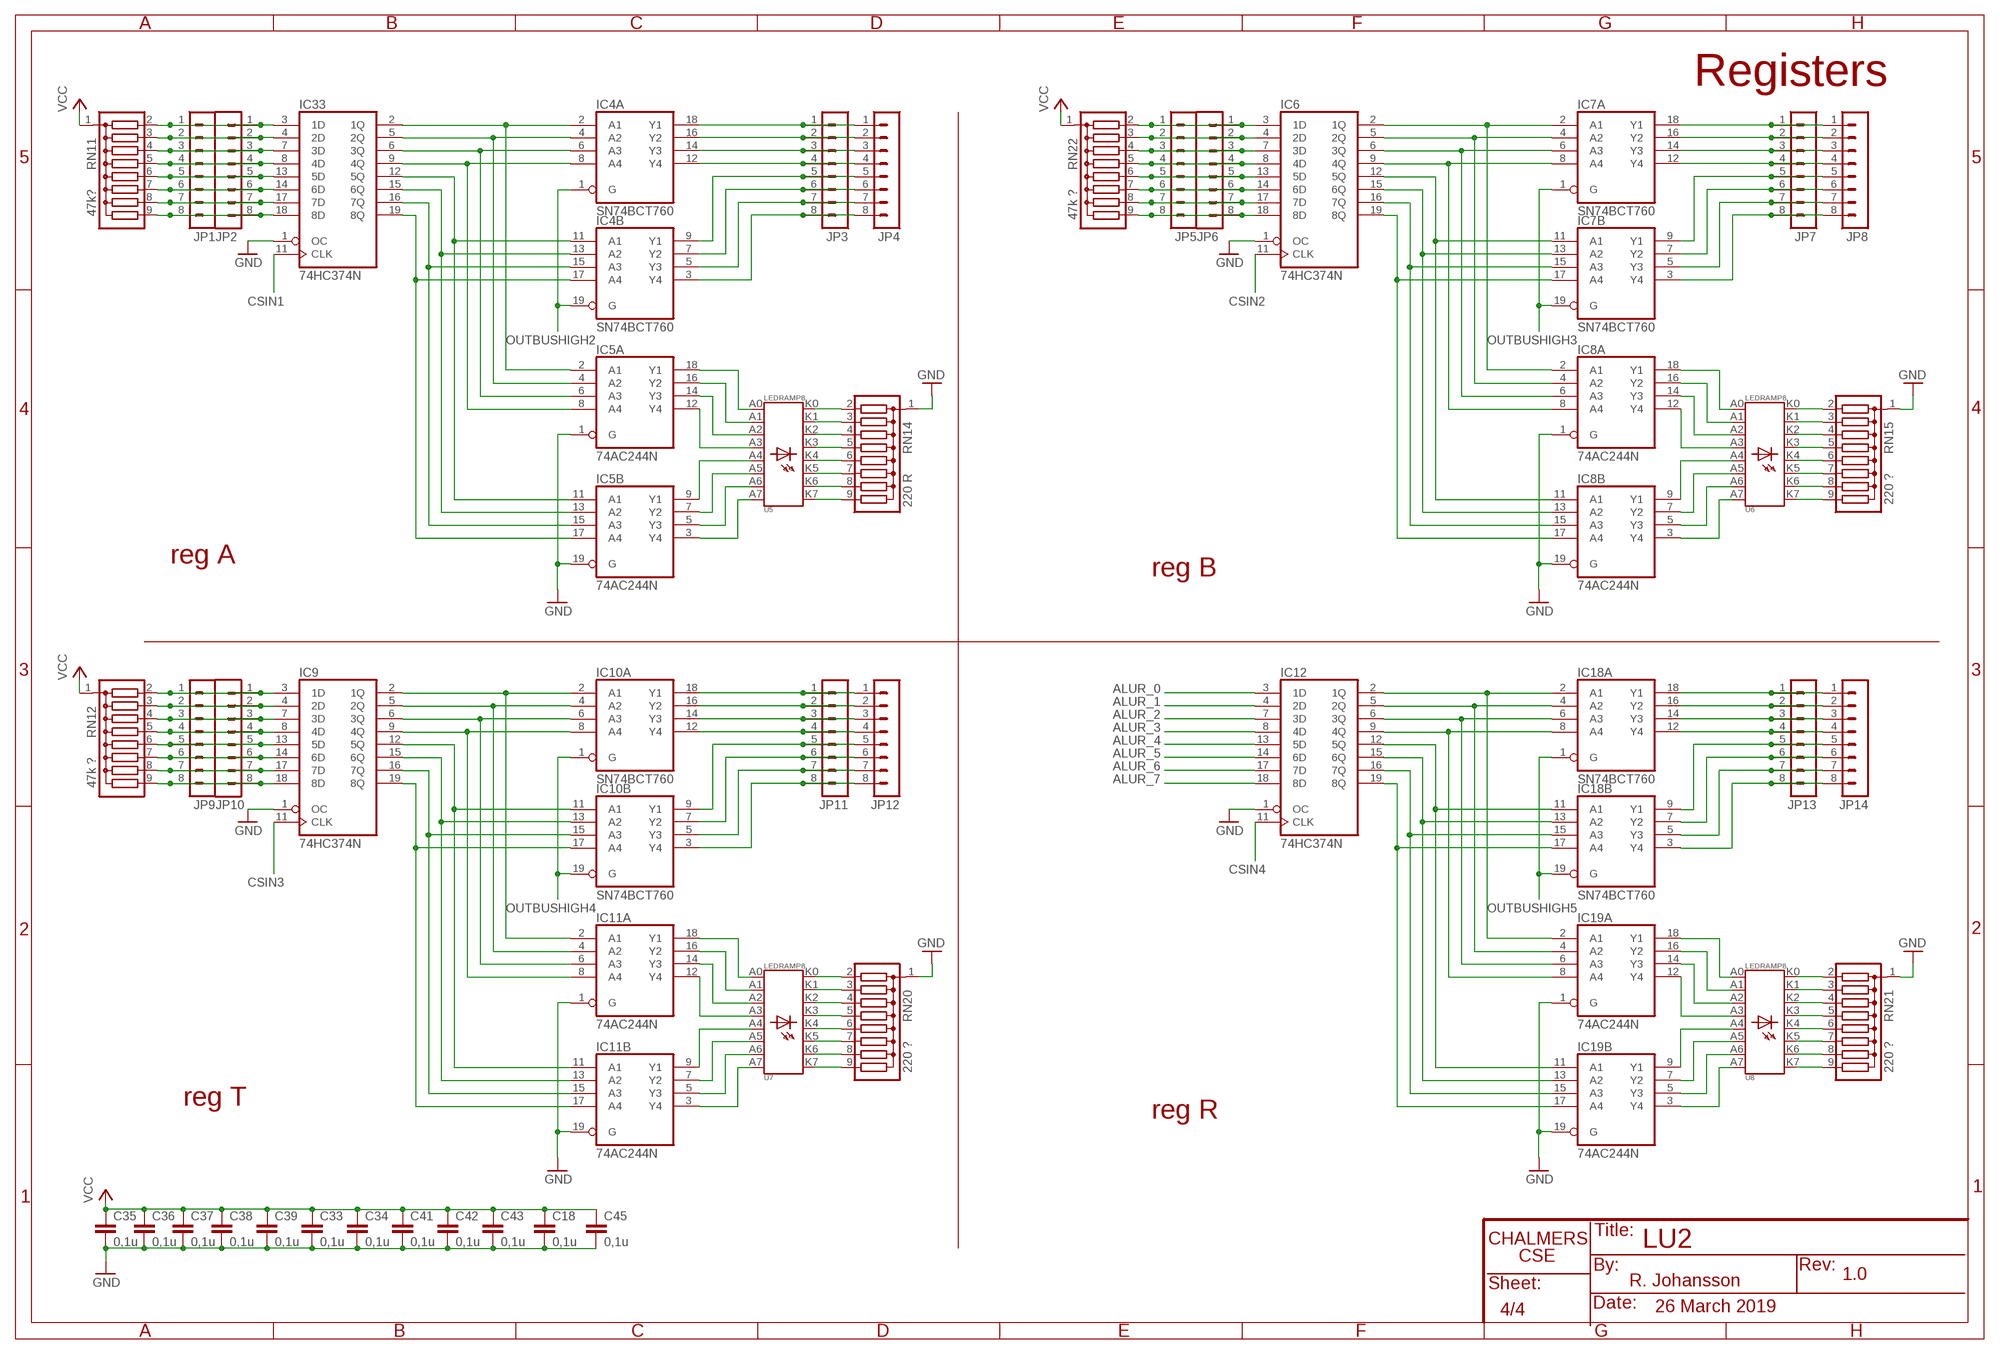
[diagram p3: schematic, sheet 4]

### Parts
C18  0,1u  C313  [C313]
C33  0,1u  C313  [C313]
C34  0,1u  C313  [C313]
C35  0,1u  C313  [C313]
C36  0,1u  C313  [C313]
C37  0,1u  C313  [C313]
C38  0,1u  C313  [C313]
C39  0,1u  C313  [C313]
C41  0,1u  C313  [C313]
C42  0,1u  C313  [C313]
C43  0,1u  C313  [C313]
C45  0,1u  C313  [C313]
IC4  SN74BCT760  74AC244N  [DIL20]
IC5  74AC244N  [DIL20]
IC6  74HC374N  [DIL20]
IC7  SN74BCT760  74AC244N  [DIL20]
IC8  74AC244N  [DIL20]
IC9  74HC374N  [DIL20]
IC10  SN74BCT760  74AC244N  [DIL20]
IC11  74AC244N  [DIL20]
IC12  74HC374N  [DIL20]
IC18  SN74BCT760  74AC244N  [DIL20]
IC19  74AC244N  [DIL20]
IC33  74HC374N  [DIL20]
JP1  MA08R-1  [MA08R-1]
JP2  MA08R-1  [MA08R-1]
JP3  MA08R-1  [MA08R-1]
JP4  MA08R-1  [MA08R-1]
JP5  MA08R-1  [MA08R-1]
JP6  MA08R-1  [MA08R-1]
JP7  MA08R-1  [MA08R-1]
JP8  MA08R-1  [MA08R-1]
JP9  MA08R-1  [MA08R-1]
JP10  MA08R-1  [MA08R-1]
JP11  MA08R-1  [MA08R-1]
JP12  MA08R-1  [MA08R-1]
JP13  MA08R-1  [MA08R-1]
JP14  MA08R-1  [MA08R-1]
RN11  47k?  SIL9  [SIL9R]
RN12  47k ?  SIL9  [SIL9R]
RN14  220 R  SIL9  [SIL9R]
RN15  220 ?  SIL9  [SIL9R]
RN20  220 ?  SIL9  [SIL9R]
RN21  220 ?  SIL9  [SIL9R]
RN22  47k ?  SIL9  [SIL9R]
U5  LEDRAMP8  [LEDRAMP8]
U6  LEDRAMP8  [LEDRAMP8]
U7  LEDRAMP8  [LEDRAMP8]
U8  LEDRAMP8  [LEDRAMP8]

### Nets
ALUR_0: IC12.3(1D) ; also sheet 3
ALUR_1: IC12.4(2D) ; also sheet 3
ALUR_2: IC12.7(3D) ; also sheet 3
ALUR_3: IC12.8(4D) ; also sheet 3
ALUR_4: IC12.13(5D) ; also sheet 3
ALUR_5: IC12.14(6D) ; also sheet 3
ALUR_6: IC12.17(7D) ; also sheet 3
ALUR_7: IC12.18(8D) ; also sheet 3
CSIN1: IC33.11(CLK) ; also sheet 1
CSIN2: IC6.11(CLK) ; also sheet 1
CSIN3: IC9.11(CLK) ; also sheet 1
CSIN4: IC12.11(CLK) ; also sheet 1
GND: C18.2 C33.2 C34.2 C35.2 C36.2 C37.2 C38.2 C39.2 C41.2 C42.2 C43.2 C45.2 IC5.1(A:G) IC5.19(B:G) IC6.1(OC) IC8.1(A:G) IC8.19(B:G) IC9.1(OC) IC11.1(A:G) IC11.19(B:G) IC12.1(OC) IC19.1(A:G) IC19.19(B:G) IC33.1(OC) RN14.1 RN15.1 RN20.1 RN21.1 ; also sheet 1,2,3
N$6: IC4.18(A:Y1) JP3.1 JP4.1
N$25: IC7.18(A:Y1) JP7.1 JP8.1
N$26: IC4.16(A:Y2) JP3.2 JP4.2
N$27: IC4.14(A:Y3) JP3.3 JP4.3
N$28: IC4.12(A:Y4) JP3.4 JP4.4
N$30: IC4.9(B:Y1) JP3.5 JP4.5
N$32: IC4.7(B:Y2) JP3.6 JP4.6
N$34: IC4.5(B:Y3) JP3.7 JP4.7
N$36: IC4.3(B:Y4) JP3.8 JP4.8
N$38: IC5.18(A:Y1) U5.A0
N$40: IC5.16(A:Y2) U5.A1
N$41: IC5.14(A:Y3) U5.A2
N$42: IC5.12(A:Y4) U5.A3
N$43: IC5.9(B:Y1) U5.A4
N$44: IC5.7(B:Y2) U5.A5
N$45: IC5.5(B:Y3) U5.A6
N$50: IC5.3(B:Y4) U5.A7
N$51: RN14.2 U5.K0(C0)
N$53: IC7.16(A:Y2) JP7.2 JP8.2
N$54: RN14.3 U5.K1(C1)
N$56: RN14.4 U5.K2(C2)
N$57: RN14.5 U5.K3(C3)
N$58: RN14.6 U5.K4(C4)
N$59: RN14.7 U5.K5(C5)
N$60: RN14.8 U5.K6(C6)
N$61: RN14.9 U5.K7(C7)
N$62: IC7.14(A:Y3) JP7.3 JP8.3
N$63: IC4.17(B:A4) IC5.17(B:A4) IC33.19(8Q)
N$64: IC4.15(B:A3) IC5.15(B:A3) IC33.16(7Q)
N$65: IC4.13(B:A2) IC5.13(B:A2) IC33.15(6Q)
N$66: IC4.11(B:A1) IC5.11(B:A1) IC33.12(5Q)
N$67: IC4.8(A:A4) IC5.8(A:A4) IC33.9(4Q)
N$68: IC4.6(A:A3) IC5.6(A:A3) IC33.6(3Q)
N$69: IC4.4(A:A2) IC5.4(A:A2) IC33.5(2Q)
N$70: IC4.2(A:A1) IC5.2(A:A1) IC33.2(1Q)
N$71: IC7.12(A:Y4) JP7.4 JP8.4
N$77: IC7.9(B:Y1) JP7.5 JP8.5
N$79: IC7.7(B:Y2) JP7.6 JP8.6
N$84: IC7.5(B:Y3) JP7.7 JP8.7
N$85: IC7.3(B:Y4) JP7.8 JP8.8
N$86: IC8.18(A:Y1) U6.A0
N$87: IC8.16(A:Y2) U6.A1
N$88: IC8.14(A:Y3) U6.A2
N$89: IC8.12(A:Y4) U6.A3
N$92: IC8.9(B:Y1) U6.A4
N$93: IC8.7(B:Y2) U6.A5
N$94: IC8.5(B:Y3) U6.A6
N$95: IC8.3(B:Y4) U6.A7
N$96: RN15.2 U6.K0(C0)
N$97: RN15.3 U6.K1(C1)
N$98: RN15.4 U6.K2(C2)
N$99: RN15.5 U6.K3(C3)
N$100: RN15.6 U6.K4(C4)
N$105: RN15.7 U6.K5(C5)
N$106: RN15.8 U6.K6(C6)
N$107: RN15.9 U6.K7(C7)
N$108: IC6.19(8Q) IC7.17(B:A4) IC8.17(B:A4)
N$109: IC6.16(7Q) IC7.15(B:A3) IC8.15(B:A3)
N$110: IC6.15(6Q) IC7.13(B:A2) IC8.13(B:A2)
N$111: IC6.12(5Q) IC7.11(B:A1) IC8.11(B:A1)
N$112: IC6.9(4Q) IC7.8(A:A4) IC8.8(A:A4)
N$113: IC6.6(3Q) IC7.6(A:A3) IC8.6(A:A3)
N$114: IC6.5(2Q) IC7.4(A:A2) IC8.4(A:A2)
N$115: IC6.2(1Q) IC7.2(A:A1) IC8.2(A:A1)
N$116: IC6.3(1D) JP5.1 JP6.1 RN22.2
N$120: IC6.4(2D) JP5.2 JP6.2 RN22.3
N$122: IC6.7(3D) JP5.3 JP6.3 RN22.4
N$123: IC6.8(4D) JP5.4 JP6.4 RN22.5
N$124: IC6.13(5D) JP5.5 JP6.5 RN22.6
N$125: IC6.14(6D) JP5.6 JP6.6 RN22.7
N$126: IC6.17(7D) JP5.7 JP6.7 RN22.8
N$127: IC6.18(8D) JP5.8 JP6.8 RN22.9
N$128: IC10.18(A:Y1) JP11.1 JP12.1
N$129: IC10.16(A:Y2) JP11.2 JP12.2
N$130: IC10.14(A:Y3) JP11.3 JP12.3
N$131: IC10.12(A:Y4) JP11.4 JP12.4
N$132: IC10.9(B:Y1) JP11.5 JP12.5
N$134: IC10.7(B:Y2) JP11.6 JP12.6
N$135: IC10.5(B:Y3) JP11.7 JP12.7
N$139: IC10.3(B:Y4) JP11.8 JP12.8
N$140: IC11.18(A:Y1) U7.A0
N$141: IC11.16(A:Y2) U7.A1
N$142: IC11.14(A:Y3) U7.A2
N$143: IC11.12(A:Y4) U7.A3
N$193: IC11.9(B:Y1) U7.A4
N$194: IC11.7(B:Y2) U7.A5
N$195: IC11.5(B:Y3) U7.A6
N$196: IC11.3(B:Y4) U7.A7
N$205: RN20.2 U7.K0(C0)
N$206: RN20.3 U7.K1(C1)
N$207: RN20.4 U7.K2(C2)
N$208: RN20.5 U7.K3(C3)
N$209: RN20.6 U7.K4(C4)
N$210: RN20.7 U7.K5(C5)
N$211: RN20.8 U7.K6(C6)
N$212: RN20.9 U7.K7(C7)
N$221: IC9.19(8Q) IC10.17(B:A4) IC11.17(B:A4)
N$222: IC9.16(7Q) IC10.15(B:A3) IC11.15(B:A3)
N$223: IC9.15(6Q) IC10.13(B:A2) IC11.13(B:A2)
N$224: IC9.12(5Q) IC10.11(B:A1) IC11.11(B:A1)
N$225: IC9.9(4Q) IC10.8(A:A4) IC11.8(A:A4)
N$226: IC9.6(3Q) IC10.6(A:A3) IC11.6(A:A3)
N$227: IC9.5(2Q) IC10.4(A:A2) IC11.4(A:A2)
N$228: IC9.2(1Q) IC10.2(A:A1) IC11.2(A:A1)
N$229: IC9.3(1D) JP9.1 JP10.1 RN12.2
N$231: IC9.4(2D) JP9.2 JP10.2 RN12.3
N$232: IC9.7(3D) JP9.3 JP10.3 RN12.4
N$233: IC9.8(4D) JP9.4 JP10.4 RN12.5
N$234: IC9.13(5D) JP9.5 JP10.5 RN12.6
N$235: IC9.14(6D) JP9.6 JP10.6 RN12.7
N$236: IC9.17(7D) JP9.7 JP10.7 RN12.8
N$237: IC9.18(8D) JP9.8 JP10.8 RN12.9
N$239: IC18.18(A:Y1) JP13.1 JP14.1
N$240: IC18.16(A:Y2) JP13.2 JP14.2
N$241: IC18.14(A:Y3) JP13.3 JP14.3
N$242: IC18.12(A:Y4) JP13.4 JP14.4
N$243: IC18.9(B:Y1) JP13.5 JP14.5
N$244: IC18.7(B:Y2) JP13.6 JP14.6
N$245: IC18.5(B:Y3) JP13.7 JP14.7
N$246: IC18.3(B:Y4) JP13.8 JP14.8
N$247: IC19.18(A:Y1) U8.A0
N$249: IC19.16(A:Y2) U8.A1
N$250: IC19.14(A:Y3) U8.A2
N$251: IC19.12(A:Y4) U8.A3
N$252: IC19.9(B:Y1) U8.A4
N$253: IC19.7(B:Y2) U8.A5
N$254: IC19.5(B:Y3) U8.A6
N$257: IC19.3(B:Y4) U8.A7
N$258: RN21.2 U8.K0(C0)
N$259: RN21.3 U8.K1(C1)
N$260: RN21.4 U8.K2(C2)
N$261: RN21.5 U8.K3(C3)
N$262: RN21.6 U8.K4(C4)
N$263: RN21.7 U8.K5(C5)
N$264: RN21.8 U8.K6(C6)
N$265: RN21.9 U8.K7(C7)
N$266: IC12.19(8Q) IC18.17(B:A4) IC19.17(B:A4)
N$267: IC12.16(7Q) IC18.15(B:A3) IC19.15(B:A3)
N$268: IC12.15(6Q) IC18.13(B:A2) IC19.13(B:A2)
N$269: IC12.12(5Q) IC18.11(B:A1) IC19.11(B:A1)
N$270: IC12.9(4Q) IC18.8(A:A4) IC19.8(A:A4)
N$271: IC12.6(3Q) IC18.6(A:A3) IC19.6(A:A3)
N$272: IC12.5(2Q) IC18.4(A:A2) IC19.4(A:A2)
N$273: IC12.2(1Q) IC18.2(A:A1) IC19.2(A:A1)
N$274: IC33.3(1D) JP1.1 JP2.1 RN11.2
N$276: IC33.4(2D) JP1.2 JP2.2 RN11.3
N$277: IC33.7(3D) JP1.3 JP2.3 RN11.4
N$278: IC33.8(4D) JP1.4 JP2.4 RN11.5
N$279: IC33.13(5D) JP1.5 JP2.5 RN11.6
N$280: IC33.14(6D) JP1.6 JP2.6 RN11.7
N$281: IC33.17(7D) JP1.7 JP2.7 RN11.8
N$282: IC33.18(8D) JP1.8 JP2.8 RN11.9
OUTBUSHIGH2: IC4.1(A:G) IC4.19(B:G) ; also sheet 1
OUTBUSHIGH3: IC7.1(A:G) IC7.19(B:G) ; also sheet 1
OUTBUSHIGH4: IC10.1(A:G) IC10.19(B:G) ; also sheet 1
OUTBUSHIGH5: IC18.1(A:G) IC18.19(B:G) ; also sheet 1
VCC: C18.1 C33.1 C34.1 C35.1 C36.1 C37.1 C38.1 C39.1 C41.1 C42.1 C43.1 C45.1 RN11.1 RN12.1 RN22.1 ; also sheet 1,2,3

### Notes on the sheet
- Registers
- reg A
- reg B
- reg T
- reg R
- LU2
- 1.0
- R. Johansson
- 26 March 2019

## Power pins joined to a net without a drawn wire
GND: IC1.12(GND) IC2.12(GND) IC3.10(GND) IC4.10(P:GND) IC5.10(P:GND) IC6.10(GND) IC7.10(P:GND) IC8.10(P:GND) IC9.10(GND) IC10.10(P:GND) IC11.10(P:GND) IC12.10(GND) IC13.10(GND) IC14.10(GND) IC15.10(GND) IC16.10(GND) IC17.10(GND) IC18.10(P:GND) IC19.10(P:GND) IC20.10(P:GND) IC21.10(P:GND) IC22.10(GND) IC23.7(P:GND) IC24.10(P:GND) IC25.10(P:GND) IC26.10(GND) IC27.10(GND) IC28.10(P:GND) IC29.10(GND) IC30.10(P:GND) IC31.10(GND) IC32.10(P:GND) IC33.10(GND) IC34.10(GND) IC35.10(P:GND) IC37.10(P:GND)
VCC: IC1.24(VCC) IC2.24(VCC) IC3.20(VCC) IC4.20(P:VCC) IC5.20(P:VCC) IC6.20(VCC) IC7.20(P:VCC) IC8.20(P:VCC) IC9.20(VCC) IC10.20(P:VCC) IC11.20(P:VCC) IC12.20(VCC) IC13.20(VCC) IC14.20(VCC) IC15.20(VCC) IC16.20(VCC) IC17.20(VCC) IC18.20(P:VCC) IC19.20(P:VCC) IC20.20(P:VCC) IC21.20(P:VCC) IC22.20(VCC) IC23.14(P:VCC) IC24.20(P:VCC) IC25.20(P:VCC) IC26.20(VCC) IC27.20(VCC) IC28.20(P:VCC) IC29.20(VCC) IC30.20(P:VCC) IC31.20(VCC) IC32.20(P:VCC) IC33.20(VCC) IC34.20(VCC) IC35.20(P:VCC) IC37.20(P:VCC)

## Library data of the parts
C1 C3 = rcl:CPOL-EU: POLARIZED CAPACITOR, European symbol
C2 C5 = rcl:C-EU: CAPACITOR, European symbol
C4 C6-C20 C24-C39 C41-C43 C45 = 0misc:C313
D1-D4 = diode:1N4004: DIODE
IC1 IC2 = 74xx-eu:74*154: 4-line to 16-line data SELECTOR/MULTIPLEXER
IC3 IC6 IC9 IC12-IC17 IC22 IC33 IC34 = 74xx-eu:74*374: Octal D type transparent LATCH, edge triggered
IC4 IC5 IC7 IC8 IC10 IC11 IC18-IC21 IC24 IC25 IC28 IC30 IC32 IC35 IC37 = 74xx-eu:74*244: Octal BUFFER and LINE DRIVER, 3-state
IC23 = 74xx-eu:74*74: Dual D type positive edge triggered FLIP FLOP, preset and clear
IC26 IC27 IC29 IC31 = 74xx-eu:74*245: Octal BUS TRANSCEIVER, 3-state
JP1-JP14 SV1-SV3 SV5-SV8 SV10-SV12 = 0misc:MA08R-1: Header round pads
LED1-LED20 = led:LED: LED
P1 = 0misc:DC21-PCB
P2 = 0misc:USB-NORMAL-S
P8 = 0misc:ARM_CONTROL: Connectors for ARM CTRL board
R1-R14 R16-R39 = rcl:R-EU_: RESISTOR, European symbol
RN1 RN3 RN5-RN12 RN14 RN15 RN20-RN24 RN26 = 0misc:SIL9
RN2 RN4 = resistor-net:RNX8: RESISTOR NETWORK; OC_FARNELL: unknown; OC_NEWARK: unknown
RN16-RN19 = resistor-dil:8R-N: DIL RESISTOR; OC_FARNELL: unknown; OC_NEWARK: unknown
S1 S2 = switch-dil:DS08: DIL/CODE SWITCH; MPN: DS08; OC_FARNELL: unknown; OC_NEWARK: 73J0071
SW1-SW6 SW8-SW17 = 0misc:ELEDIS_TOGGLE_MINIATURE
SW7 = 0misc:ELEDIS_TOGGLE_MINIATURE_MOM
U1 = 0misc:LM1117
U5-U11 = 0misc:LEDRAMP8
U13-U16 = 0misc:LED7_CA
